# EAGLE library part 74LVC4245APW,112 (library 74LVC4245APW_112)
74LVC4245A - Octal dual supply translating transceiver; 3-state@en-us Source: Datasheet
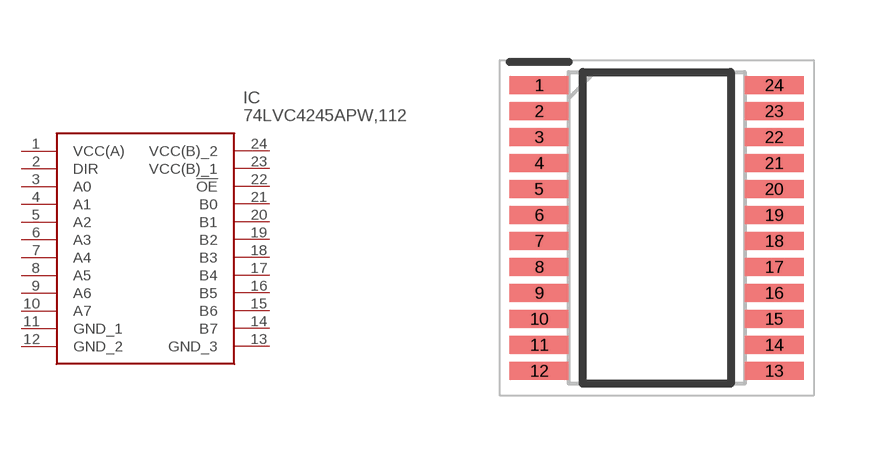
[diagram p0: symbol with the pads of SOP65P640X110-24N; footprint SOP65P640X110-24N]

Designator prefix IC

## 74LVC4245APW,112 (Arrow_Part_Number: 74LVC4245APW,112; Arrow_Price-Stock: https://www.arrow.com/en/products/74lvc4245apw112/nexperia; Description: 74LVC4245A - Octal dual supply translating transceiver; 3-state@en-us; Height: 1.1mm; Manufacturer_Name: Nexperia; Manufacturer_Part_Number: 74LVC4245APW,112; Mouser_Part_Number: 771-LVC4245APW112; Mouser_Price-Stock: https://www.mouser.co.uk/ProductDetail/Nexperia/74LVC4245APW112?qs=me8TqzrmIYVuB5bh8j1Vew%3D%3D)  [SOP65P640X110-24N]
1  VCC(A)
2  DIR
3  A0
4  A1
5  A2
6  A3
7  A4
8  A5
9  A6
10  A7
11  GND_1
12  GND_2
13  GND_3
14  B7
15  B6
16  B5
17  B4
18  B3
19  B2
20  B1
21  B0
22  !OE
23  VCC(B)_1
24  VCC(B)_2

## Footprint SOP65P640X110-24N (pad centres in mm)
SOT355-1
smd 1.475 x 0.45: 1 -2.938,3.575; 2 -2.938,2.925; 3 -2.938,2.275; 4 -2.938,1.625; 5 -2.938,0.975; 6 -2.938,0.325; 7 -2.938,-0.325; 8 -2.938,-0.975; 9 -2.938,-1.625; 10 -2.938,-2.275; 11 -2.938,-2.925; 12 -2.938,-3.575; 13 2.938,-3.575; 14 2.938,-2.925; 15 2.938,-2.275; 16 2.938,-1.625; 17 2.938,-0.975; 18 2.938,-0.325; 19 2.938,0.325; 20 2.938,0.975; 21 2.938,1.625; 22 2.938,2.275; 23 2.938,2.925; 24 2.938,3.575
